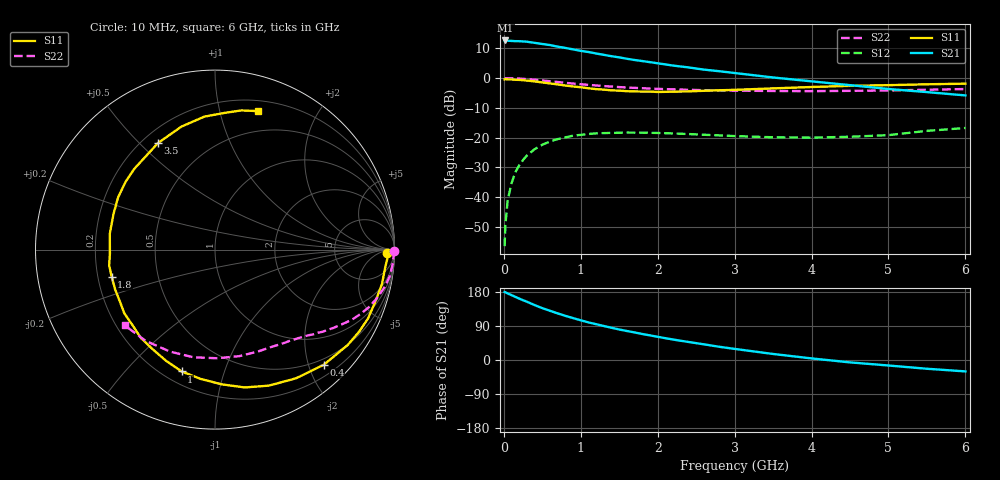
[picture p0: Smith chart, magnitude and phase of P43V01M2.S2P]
! SIEMENS Small Signal Semiconductors
! BFP182
! Si NPN RF Bipolar Junction Transistor in SOT143
! VCE = 3 V  IC = 1.2 mA
! Common Emitter S-Parameters:  March  1996
# GHz  S  MA  R  50
!  f  S11  S21  S12  S22
! GHz  MAG  ANG  MAG  ANG  MAG  ANG  MAG  ANG
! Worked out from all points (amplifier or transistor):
!   36 points, 10 MHz to 6 GHz, reference 50 ohm
!   highest |S21| = 12.7 dB at 20 MHz (marker M1)
!   |S21| within 3 dB of that: start of sweep to 898.9 MHz
!   unconditionally stable (mu >= 1): 2.528 GHz to end of sweep
!   at 250 MHz: K = 0.10, MSG = 19.9 dB, |S12| = -27.5 dB
!   at 1.4 GHz: K = 0.56, MSG = 12.9 dB, |S12| = -18.4 dB
!   at 6 GHz: K = 1.03, MAG = 4.3 dB, |S12| = -16.7 dB
!   S11 on the Smith chart (normalised r, x): 10 MHz: 38, -16; 400 MHz: 0.39, -2.27; 1 GHz: 0.27, -0.73; 1.8 GHz: 0.26, -0.12; 3.5 GHz: 0.26, +0.57; 6 GHz: 0.30, +1.32
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0.01  0.9563 -1.1  4.254 179.4  0.0015 83.9  0.9982 -0.4
0.02  0.9628 -2.6  4.304 178.8  0.0034 87.2  0.9947 -0.9
0.05  0.9532 -6.2  4.26 175.6  0.0089 90.2  0.9959 -2.2
0.1  0.9498 -11.7  4.227 171.2  0.0172 81.2  0.9931 -4.5
0.15  0.9393 -18.0  4.189 166.6  0.0262 78.7  0.9886 -6.8
0.2  0.935 -24.2  4.183 162.0  0.0344 75.3  0.9835 -8.9
0.3  0.9107 -35.7  4.099 153.8  0.0501 68.4  0.9637 -13.1
0.4  0.8828 -46.6  3.924 144.9  0.0639 61.7  0.9407 -16.9
0.5  0.8474 -57.8  3.755 136.9  0.0761 55.5  0.9156 -20.5
0.6  0.8152 -68.4  3.603 129.8  0.0863 49.8  0.8873 -23.8
0.8  0.7517 -87.1  3.224 116.5  0.1012 39.6  0.8342 -29.2
1  0.7039 -105.3  2.876 104.8  0.1115 31.7  0.7907 -33.5
1.1  0.6764 -113.9  2.755 99.2  0.1154 28.2  0.7711 -35.4
1.3  0.6423 -130.1  2.464 89.7  0.1193 21.9  0.7365 -39.0
1.5  0.6177 -144.8  2.235 80.5  0.1207 16.9  0.7082 -42.3
1.8  0.5951 -165.2  1.939 68.6  0.1213 11.3  0.6782 -46.6
2.2  0.5928 171.4  1.628 54.0  0.1177 5.5  0.6493 -52.9
2.8  0.6255 142.5  1.309 34.9  0.1092 1.4  0.6207 -63.1
3.5  0.6734 118.1  1.027 15.9  0.1015 2.4  0.6089 -77.2
4.5  0.7432 94.6  0.763 -6.3  0.1036 10.3  0.612 -101.3
5.5  0.7892 79.3  0.583 -23.1  0.13 16.7  0.6386 -127.3
6  0.8081 72.7  0.513 -30.1  0.1455 15.0  0.6568 -140.0
